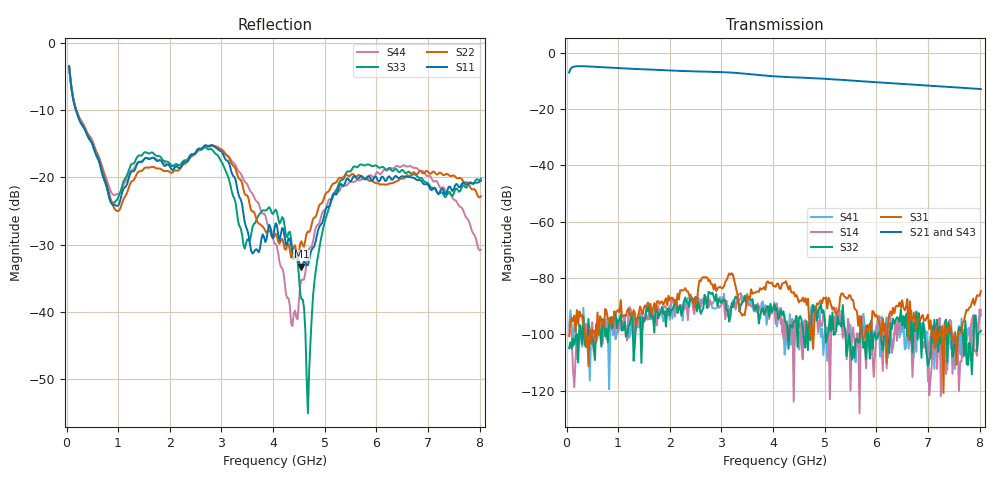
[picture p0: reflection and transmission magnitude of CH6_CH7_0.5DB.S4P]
!Agilent Technologies,E5071C,MY46316741,A.11.02
!Date: Mon Jun 01 10:33:24 2026
!Data & Calibration Information:
!1:CH6 INPUT 2:CH6 OUTPUT 3:CH7 INPUT 4:CH7 OUTPUT
!Freq	S11:SOLT4(ON)	S12:SOLT4(ON)	S13:SOLT4(ON)	S14:SOLT4(ON)
!	S21:SOLT4(ON)	S22:SOLT4(ON)	S23:SOLT4(ON)	S24:SOLT4(ON)
!	S31:SOLT4(ON)	S32:SOLT4(ON)	S33:SOLT4(ON)	S34:SOLT4(ON)
!	S41:SOLT4(ON)	S42:SOLT4(ON)	S43:SOLT4(ON)	S44:SOLT4(ON)
!PortZ  Port1:50+j0  Port2:50+j0  Port3:50+j0  Port4:50+j0
!Above PortZ is port z conversion or system Z0 setting when saving the data.
!When reading, reference impedance value at option line is always used.
# Hz S dB R 50
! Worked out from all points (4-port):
!   320 points, 50 MHz to 8.025 GHz, reference 50 ohm
!   strongest paths, dB at 50 MHz, 2.05 GHz, 4.05 GHz, 6.05 GHz, 8.025 GHz:
!     S21: -7.0, -6.3, -8.3, -10.5, -12.8
!     S43: -6.9, -6.2, -8.4, -10.6, -12.9
!     S31: -100.6, -87.0, -83.2, -95.2, -84.7
!     S32: -105.0, -91.4, -91.6, -99.5, -98.7
!     S14: -98.3, -87.2, -96.3, -93.4, -93.3
!     S41: -97.3, -94.4, -90.3, -96.6, -91.5
!   lowest |S11| = -33.3 dB at 4.55 GHz (marker M1), VSWR 1.04, Z = 49.6 - j2.11 ohm
!   |S11| at or under -10 dB: 181.9 MHz to end of sweep
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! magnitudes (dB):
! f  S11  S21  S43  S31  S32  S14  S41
! 50 MHz  -3.5  -7.0  -6.9  -100.6  -105.0  -98.3  -97.3
! 950 MHz  -24.2  -5.4  -5.4  -92.4  -92.4  -95.1  -101.8
! 2.8 GHz  -15.3  -6.7  -6.7  -82.2  -85.7  -89.5  -88.5
! 4.55 GHz  -33.3  -8.8  -8.9  -88.1  -94.9  -104.8  -95.9
! 4.675 GHz  -33.1  -8.9  -9.0  -87.4  -105.6  -99.1  -100.2
! 5.425 GHz  -20.2  -9.7  -9.7  -87.3  -107.8  -108.9  -100.6
! 8.025 GHz  -20.5  -12.8  -12.9  -84.7  -98.7  -93.3  -91.5
